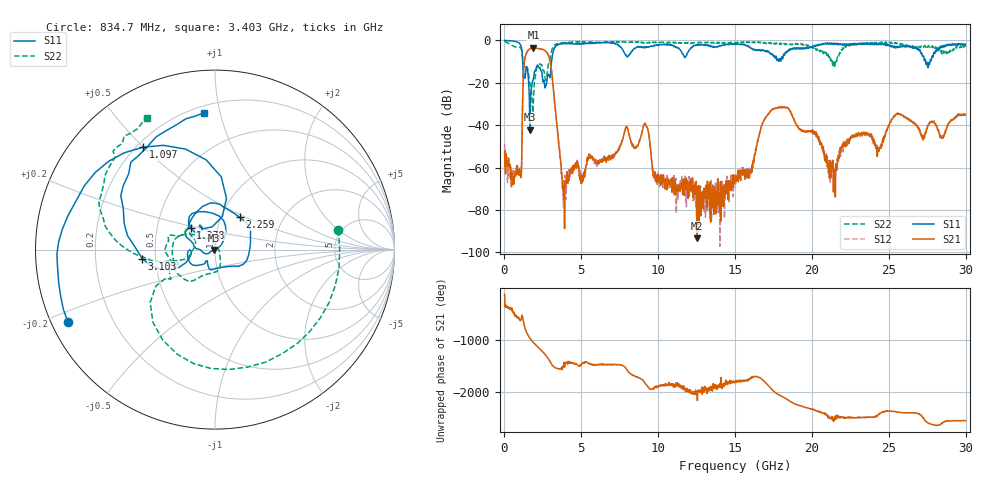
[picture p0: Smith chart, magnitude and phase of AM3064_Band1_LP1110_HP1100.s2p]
# Hz S DB R 50.0
!freq dBS11 angS11 dBS21 angS21 dBS12 angS12 dBS22 angS22
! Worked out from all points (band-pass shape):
!   1600 points, 10 MHz to 29.98 GHz, reference 50 ohm
!   highest |S21| = -3.50 dB at 1.884 GHz (marker M1); lowest = -93.4 dB at 12.53 GHz (marker M2)
!   |S21| within 3 dB of the highest: 1.404 GHz to 2.822 GHz (1.418 GHz wide, 67.1 % of centre)
!   lowest |S11| = -42.1 dB at 1.659 GHz (marker M3), VSWR 1.02, Z = 49.3 - j0.32 ohm
!   |S11| at or under -10 dB: 1.186 GHz to 3.064 GHz (1.877 GHz wide, 88.3 % of centre); 27.4 GHz to 27.68 GHz (282.9 MHz wide, 1.03 % of centre)
!   |S22| runs from -34.1 to -0.4 dB; largest |S21 - S12| = 0.0088
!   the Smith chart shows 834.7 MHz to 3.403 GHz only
!   S11 on the Smith chart (normalised r, x): 834.7 MHz: 0.05, -0.23; 1.097 GHz: 0.22, +0.50; 1.378 GHz: 0.74, +0.19; 2.259 GHz: 1.22, +0.46; 3.103 GHz: 0.42, -0.05; 3.403 GHz: 0.24, +0.90
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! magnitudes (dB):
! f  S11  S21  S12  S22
! 10 MHz  0.0  -52.5  -48.7  -0.4
! 834.7 MHz  -0.8  -63.0  -60.9  -3.2
! 1.097 GHz  -3.1  -63.4  -62.4  -4.2
! 1.378 GHz  -14.8  -7.0  -7.0  -12.8
! 1.659 GHz  -42.1  -4.0  -3.9  -20.7
! 1.884 GHz  -18.0  -3.5  -3.5  -27.6
! 2.259 GHz  -12.9  -4.0  -3.9  -11.5
! 3.103 GHz  -7.8  -16.9  -17.1  -4.1
! 3.403 GHz  -2.3  -39.2  -39.3  -1.7
! 3.871 GHz  -1.4  -69.0  -74.1  -1.1
! 5.015 GHz  -1.5  -67.4  -66.9  -0.6
! 9.157 GHz  -3.5  -39.4  -39.0  -1.1
! 10 GHz  -2.2  -63.7  -62.5  -0.9
! 12.53 GHz  -2.2  -93.4  -70.9  -1.0
! 15 GHz  -1.8  -64.8  -63.8  -1.2
! 17.46 GHz  -6.9  -32.6  -32.4  -1.3
! 19.99 GHz  -3.4  -43.0  -43.0  -3.0
! 21.38 GHz  -1.3  -57.5  -59.4  -11.1
! 22.58 GHz  -1.5  -46.0  -45.3  -2.2
! 24.38 GHz  -1.6  -51.2  -51.2  -1.4
! 25 GHz  -2.0  -40.0  -40.4  -1.2
! 29.98 GHz  -1.7  -35.0  -35.1  -3.0
